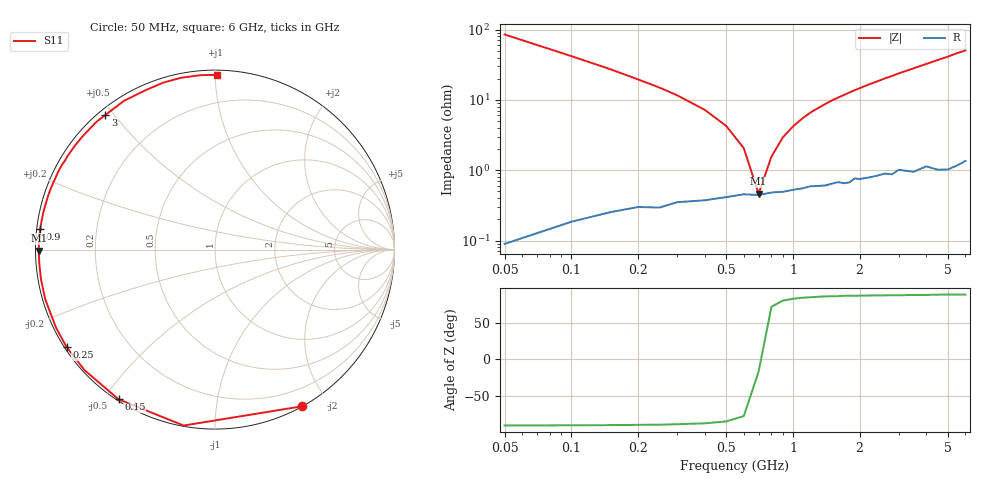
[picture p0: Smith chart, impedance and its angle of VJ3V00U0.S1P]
! Infineon Technologies  Discrete & RF Semiconductors
! BB 914
! Si Tuning Diode in SOT23
! VR = 3 V
! S-Parameters:  July  1999
# GHz  S  MA  R  50
!  f  S11
! GHz  MAG  ANG
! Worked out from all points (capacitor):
!   34 points, 50 MHz to 6 GHz, reference 50 ohm
!   read as one part to ground: C = 37.2 pF near 50 MHz
!   lowest |Z| = 463 mohm at 700 MHz (marker M1)
!   series resonance near 708.1 MHz, so ESL is about 1.4 nH
!   S11 on the Smith chart (normalised r, x): 50 MHz: 0.00, -1.70; 150 MHz: 0.01, -0.55; 250 MHz: 0.01, -0.30; 900 MHz: 0.01, +0.06; 3 GHz: 0.02, +0.47; 6 GHz: 0.03, +1.01
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0.05  0.9991 -60.9
0.1  0.9957 -100.1
0.15  0.9922 -122.8
0.2  0.9897 -137.3
0.25  0.9892 -146.7
0.3  0.9868 -153.8
0.4  0.9855 -163.6
0.5  0.9837 -170.3
0.6  0.982 -175.4
0.7  0.9824 -179.7
0.8  0.9809 176.6
0.9  0.9805 173.4
1.2  0.977 165.0
1.5  0.9755 157.8
1.6  0.9744 155.7
1.7  0.9755 153.6
1.9  0.9719 149.3
2.2  0.9719 143.4
2.4  0.9709 139.8
2.6  0.9697 136.0
2.8  0.9711 132.8
3  0.9675 129.2
3.5  0.9715 121.4
4  0.9686 114.0
4.5  0.974 107.2
5  0.9758 101.1
5.5  0.9751 94.7
6  0.9735 89.5
